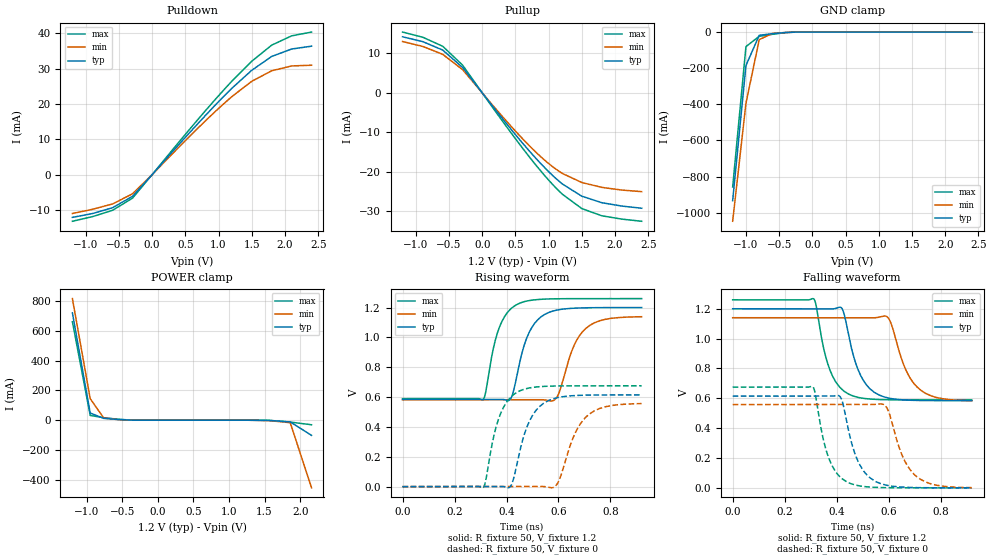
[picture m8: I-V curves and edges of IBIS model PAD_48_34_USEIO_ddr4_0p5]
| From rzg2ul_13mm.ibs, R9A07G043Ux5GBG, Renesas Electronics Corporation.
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[Model] PAD_48_34_USEIO_ddr4_0p5
Model_type I/O
Polarity   Non-Inverting
Vinl = 0.5070
Vinh = 0.6930
Vmeas= 0.600
| Capacitance   typ   min   max
C_comp   2.102e-12   2.013e-12   2.214e-12
[Model Spec]
| Subparameter   typ   min   max
Vmeas   0.600   0.570   0.630
Vinh   0.6930   0.6630   0.7230
Vinl   0.5070   0.4770   0.5370
| Variables   typ   min   max
[GND Clamp Reference]   0   0   0
[POWER Clamp Reference]   1.2   1.14   1.26
[Pulldown Reference]   0   0   0
[Pullup Reference]   1.2   1.14   1.26
[Temperature Range]   25   125   -40
[Voltage Range]   1.2   1.14   1.26
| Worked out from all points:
|   slope of the pulldown table from 0 to 0.18 V, typ, clamps not added: 47.1 ohm
|   slope of the pullup table from 0 to 0.18 V, typ, clamps not added: 46.4 ohm
|   GND clamp passes 1 mA (typ) near -0.30 V on its own axis
|   POWER clamp passes 1 mA (typ) near -0.38 V on its own axis
|   rising waveform, R_fixture 50, V_fixture 1.2: 20-80 % time 65.5ps typ, 73.3ps min, 59.2ps max; typ from 0.584 V to 1.2 V
|   rising waveform, R_fixture 50, V_fixture 0: 20-80 % time 69ps typ, 78.8ps min, 61.9ps max; typ from 0 V to 0.615 V
|   falling waveform, R_fixture 50, V_fixture 1.2: 20-80 % time 67.7ps typ, 76.9ps min, 61.8ps max; typ from 1.2 V to 0.584 V
|   falling waveform, R_fixture 50, V_fixture 0: 20-80 % time 66.6ps typ, 75.4ps min, 60.6ps max; typ from 0.614 V to 0 V
[GND Clamp]
| Voltage   I(typ)   I(min)   I(max)
-1.2V     -932.7mA   -1.047A    -857.4mA
-1V       -185.5mA   -394.3mA   -80.64mA
-800mV    -17.89mA   -41.9mA    -23.65mA
-600mV    -9.04mA    -7.411mA   -12.44mA
-400mV    -2.454mA   -2.378mA   -3.185mA
2.4V      0A         0A         0A
[POWER Clamp]
| Voltage   I(typ)   I(min)   I(max)
-1.2V     719.7mA    815.2mA    660.1mA
-950mV    48.1mA     144.6mA    32.07mA
-760mV    12.41mA    14.91mA    17.11mA
-360mV    527.4uA    791.2uA    575.5uA
1.26V     -115.5nA   -12.89uA   -796.6pA
1.56V     -1.53mA    -2.776mA   -549.4uA
1.86V     -11.39mA   -16.33mA   -12.44mA
2.16V     -101.5mA   -453.2mA   -30.39mA
[Pulldown]
| Voltage   I(typ)   I(min)   I(max)
-1.2V     -12.1mA    -11mA      -13.2mA
-895mV    -11mA      -9.8mA     -11.87mA
-595mV    -9.361mA   -8.288mA   -10.09mA
-295mV    -6.128mA   -5.421mA   -6.652mA
450mV     9.52mA     8.682mA    10.28mA
905mV     18.81mA    17.08mA    20.33mA
1.21V     24.63mA    22.25mA    26.67mA
1.5V      29.57mA    26.45mA    32.13mA
1.8V      33.49mA    29.43mA    36.69mA
2.1V      35.59mA    30.8mA     39.32mA
2.4V      36.4mA     31mA       40.4mA
[Pullup]
| Voltage   I(typ)   I(min)   I(max)
-1.2V     14.2mA     13mA       15.4mA
-895mV    12.97mA    11.76mA    14.08mA
-595mV    10.84mA    9.754mA    11.8mA
-295mV    6.423mA    5.87mA     7.012mA
300mV     -6.422mA   -5.908mA   -7.039mA
650mV     -13.56mA   -12.36mA   -14.93mA
955mV     -19.19mA   -17.26mA   -21.23mA
1.21V     -23.1mA    -20.43mA   -25.71mA
1.5V      -26.16mA   -22.69mA   -29.29mA
1.8V      -27.8mA    -23.92mA   -31.11mA
2.1V      -28.65mA   -24.6mA    -31.95mA
2.4V      -29.2mA    -25mA      -32.5mA
[Ramp]
dV/dt_r   0.3694/6.554e-11   0.3342/7.334e-11   0.4023/5.923e-11
dV/dt_f   0.3687/6.656e-11   0.3340/7.536e-11   0.4050/6.059e-11
R_load= 50
[Rising Waveform]
R_fixture = 50
V_fixture = 1.2
V_fixture_min = 1.14
V_fixture_max = 1.26
| Time   V(typ)   V(min)   V(max)
0s        584.4mV    581.7mV    589.5mV
310ps     584.4mV    581.7mV    583.4mV
363ps     584.8mV    581.7mV    1.019V
409ps     577.3mV    581.7mV    1.178V
486ps     1.029V     581.7mV    1.246V
580ps     1.177V     576.3mV    1.258V
604ps     1.187V     637.9mV    1.259V
658ps     1.196V     938.4mV    1.26V
700ps     1.198V     1.052V     1.26V
920ps     1.2V       1.139V     1.26V
[Rising Waveform]
R_fixture = 50
V_fixture = 0
V_fixture_min = 0
V_fixture_max = 0
| Time   V(typ)   V(min)   V(max)
0s        106.5nV    4.439uV    18.18nV
310ps     282.3nV    4.298uV    -6.86mV
361ps     338.8uV    4.044uV    406.7mV
412ps     -4.476mV   15.49uV    591.8mV
491ps     448.9mV    33.7uV     662.5mV
579ps     588.2mV    -6.451mV   674mV
604ps     599.4mV    49.49mV    674.8mV
662ps     610.4mV    351mV      675.5mV
708ps     613.2mV    470.1mV    675.6mV
920ps     614.8mV    556.6mV    675.7mV
[Falling Waveform]
R_fixture = 50
V_fixture = 1.2
V_fixture_min = 1.14
V_fixture_max = 1.26
| Time   V(typ)   V(min)   V(max)
0s        1.2V       1.14V      1.26V
312ps     1.2V       1.14V      1.266V
364ps     1.2V       1.14V      841.2mV
417ps     1.208V     1.14V      665.7mV
491ps     757.7mV    1.14V      603.2mV
589ps     606.3mV    1.151V     590.4mV
610ps     598.1mV    1.098V     589.8mV
664ps     588.5mV    799.1mV    589.2mV
708ps     585.7mV    678.3mV    589mV
920ps     584mV      583.4mV    588.9mV
[Falling Waveform]
R_fixture = 50
V_fixture = 0
V_fixture_min = 0
V_fixture_max = 0
| Time   V(typ)   V(min)   V(max)
0s        614.4mV    558mV      675.1mV
308ps     614.4mV    558mV      677.8mV
357ps     614.2mV    558mV      267.8mV
410ps     616.2mV    558mV      78.67mV
483ps     175.2mV    557.9mV    14.59mV
579ps     23.16mV    560mV      1.535mV
600ps     14.54mV    511.5mV    939.4uV
658ps     4.301mV    194.4mV    269.8uV
700ps     1.697mV    87.28mV    82.37uV
920ps     11.92uV    1.303mV    348.5nV
[Add Submodel]
| Submodel Name Mode
PAD_48_34_0p5_T Non-Driving
